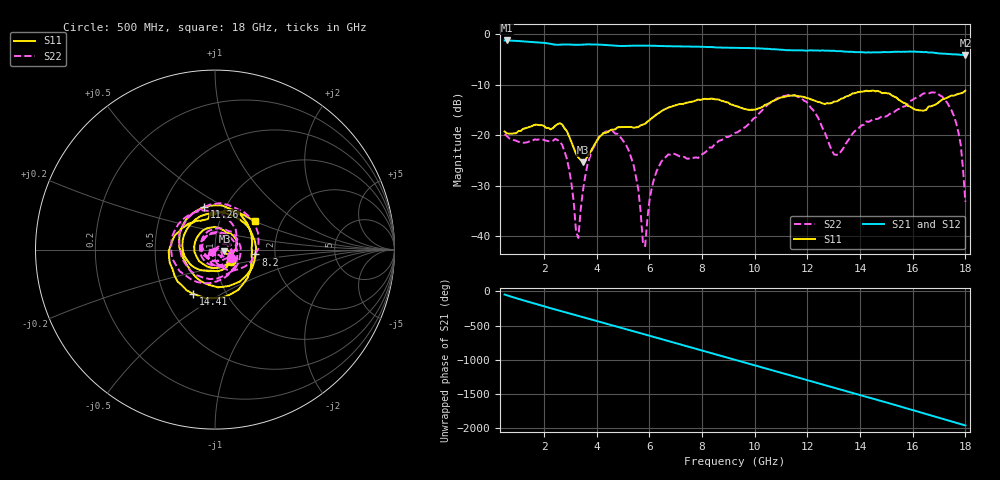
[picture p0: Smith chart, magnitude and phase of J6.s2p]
!Agilent Technologies,N5230A,MY45001360,A.07.50.67
!Agilent N5230A: A.07.50.67
!Date: Tuesday, April 16, 2024 16:00:02
!Correction: S11(Full 2 Port(1,2))
!S21(Full 2 Port(1,2))
!S12(Full 2 Port(1,2))
!S22(Full 2 Port(1,2))
!S2P File: Measurements: S11, S21, S12, S22:
# Hz S  dB  R 50
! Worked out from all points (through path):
!   201 points, 500 MHz to 18 GHz, reference 50 ohm
!   highest |S21| = -1.23 dB at 587.5 MHz (marker M1); lowest = -4.1 dB at 18 GHz (marker M2)
!   group delay of S21, straight-line fit = 302 ps
!   lowest |S11| = -25.4 dB at 3.475 GHz (marker M3), VSWR 1.11, Z = 55.6 - j1.1 ohm
!   |S11| at or under -10 dB: start of sweep to end of sweep
!   |S22| runs from -42.0 to -11.5 dB; largest |S21 - S12| = 0.0092
!   S11 on the Smith chart (normalised r, x): 500 MHz: 1.18, -0.15; 8.2 GHz: 1.58, -0.09; 11.26 GHz: 0.80, +0.40; 14.41 GHz: 0.70, -0.38; 18 GHz: 1.48, +0.51
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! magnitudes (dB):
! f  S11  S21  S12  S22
! 500 MHz  -19.3  -1.2  -1.2  -19.8
! 587.5 MHz  -19.7  -1.2  -1.2  -20.2
! 2.6 GHz  -17.6  -2.1  -2.1  -21.3
! 2.95 GHz  -20.3  -2.0  -2.0  -26.8
! 3.3 GHz  -24.4  -2.1  -2.1  -40.4
! 3.475 GHz  -25.4  -2.1  -2.0  -31.0
! 4.088 GHz  -20.5  -2.0  -2.1  -20.4
! 4.787 GHz  -18.5  -2.3  -2.3  -19.8
! 5.4 GHz  -18.5  -2.3  -2.2  -26.0
! 5.838 GHz  -17.7  -2.2  -2.2  -42.0
! 6.013 GHz  -17.0  -2.3  -2.3  -32.6
! 6.362 GHz  -15.6  -2.3  -2.3  -26.2
! 8.2 GHz  -12.9  -2.5  -2.5  -23.0
! 9.25 GHz  -14.2  -2.7  -2.7  -19.6
! 11.26 GHz  -12.2  -3.2  -3.1  -12.0
! 12.22 GHz  -13.1  -3.2  -3.2  -15.1
! 13.01 GHz  -13.3  -3.3  -3.3  -23.8
! 14.41 GHz  -11.2  -3.6  -3.6  -17.1
! 15.11 GHz  -11.8  -3.6  -3.5  -15.8
! 17.12 GHz  -13.0  -3.8  -3.9  -12.4
! 17.74 GHz  -11.8  -4.0  -4.0  -19.5
! 18 GHz  -11.2  -4.1  -4.1  -33.2
